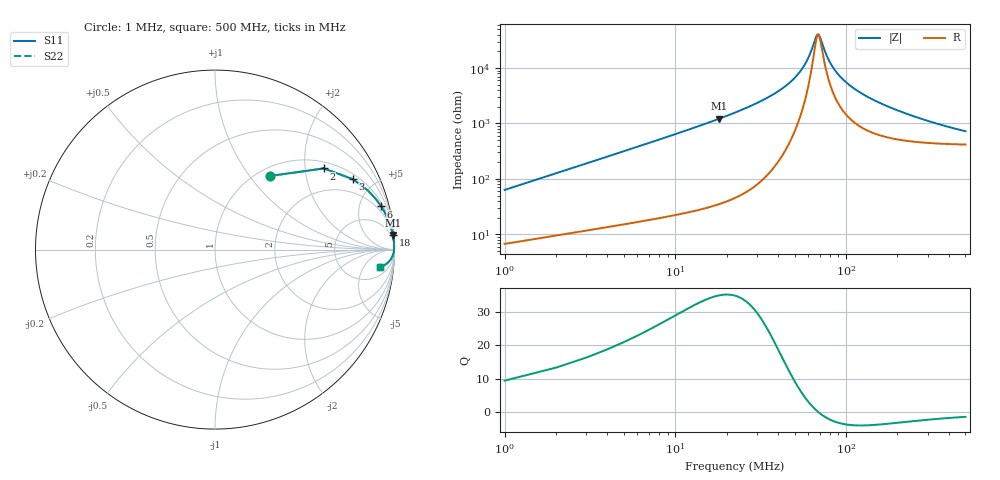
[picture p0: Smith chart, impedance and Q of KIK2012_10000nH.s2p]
!version-2
!date-01.2022
!Series
# MHz S RI R 50
!Freq ReS11 ImS11 ReS21 ImS21 ReS12 ImS12 ReS22 ImS22
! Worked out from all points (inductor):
!   500 points, 1 MHz to 500 MHz, reference 50 ohm
!   read as one part in series: L = 10 uH near 3 MHz
!   highest Q = 34.6 at 18 MHz (marker M1), where L = 10.7 uH
!   self-resonance near 68 MHz
!   S11 on the Smith chart (normalised r, x): 1 MHz: 1.13, +1.26; 2 MHz: 1.19, +2.52; 3 MHz: 1.23, +3.78; 6 MHz: 1.33, +7.60; 18 MHz: 2, +24; 500 MHz: 9, -12
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1  0.3042 0.4098  0.6958 -0.4098  0.6958 -0.4098  0.3042 0.4098
2  0.6062 0.4523  0.3938 -0.4523  0.3938 -0.4523  0.6062 0.4523
3  0.7681 0.3924  0.2319 -0.3924  0.2319 -0.3924  0.7681 0.3924
4  0.8516 0.3298  0.1484 -0.3298  0.1484 -0.3298  0.8516 0.3298
6  0.9261 0.2405  0.0739 -0.2405  0.0739 -0.2405  0.9261 0.2405
11  0.9762 0.1368  0.0238 -0.1368  0.0238 -0.1368  0.9762 0.1368
18  0.991 0.0813  0.00903 -0.0813  0.00903 -0.0813  0.991 0.0813
52  0.9981 0.013  0.00186 -0.013  0.00186 -0.013  0.9981 0.013
59  0.998 0.00705  0.00202 -0.00705  0.00202 -0.00705  0.998 0.00705
66  0.9977 0.00189  0.00231 -0.00189  0.00231 -0.00189  0.9977 0.00189
68  0.9976 0.000523  0.00241 -0.000523  0.00241 -0.000523  0.9976 0.000523
70  0.9975 -0.0008  0.00252 0.0008  0.00252 0.0008  0.9975 -0.0008
78  0.997 -0.00573  0.00305 0.00573  0.00305 0.00573  0.997 -0.00573
85  0.9964 -0.00967  0.00359 0.00967  0.00359 0.00967  0.9964 -0.00967
97  0.9953 -0.0158  0.00468 0.0158  0.00468 0.0158  0.9953 -0.0158
114  0.9935 -0.0235  0.00652 0.0235  0.00652 0.0235  0.9935 -0.0235
137  0.9905 -0.0327  0.00949 0.0327  0.00949 0.0327  0.9905 -0.0327
168  0.9858 -0.0435  0.0142 0.0435  0.0142 0.0435  0.9858 -0.0435
251  0.9701 -0.0661  0.0299 0.0661  0.0299 0.0661  0.9701 -0.0661
334  0.9521 -0.0814  0.0479 0.0814  0.0479 0.0814  0.9521 -0.0814
417  0.9339 -0.0909  0.0661 0.0909  0.0661 0.0909  0.9339 -0.0909
500  0.9168 -0.0958  0.0832 0.0958  0.0832 0.0958  0.9168 -0.0958
